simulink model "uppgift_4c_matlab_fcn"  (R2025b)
settings: Solver=VariableStepAuto  StartTime=0.0  StopTime=10.0  RelTol=1e-3
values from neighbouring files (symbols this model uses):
  AFs = 14.6    [Lektion_2.m]
  eta_vol = 0.8    [Lektion_2.m]
  m_dot_a_end = 18*1e-3    (= 0.018)    [Lektion_2.m]
  m_dot_a_start = 12*1e-3    (= 0.012)    [Lektion_2.m]
  m_dot_fi_start = m_dot_a_start/AFs    (= 0.000821917808219)    [Lektion_2.m]
  m_th_1 = 12/1000    (= 0.012)    [Lektion_2.m]
  n_cyl = 4    [Lektion_2.m]
  N_init = 3000/60    (= 50)    [Lektion_2.m]
  n_r = 2    [Lektion_2.m]
  R = 280    [Lektion_2.m]
  T_i = 320    [Lektion_2.m]
  tau_th = 1/0.1    (= 10)    [Lektion_2.m]
  V_d = 0.55/1e3    (= 0.00055)    [Lektion_2.m]
  V_i = 2/1e3    (= 0.002)    [Lektion_2.m]
undefined symbols (not defined in the file or in its folder): p_im

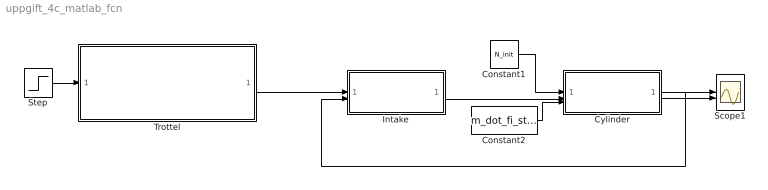
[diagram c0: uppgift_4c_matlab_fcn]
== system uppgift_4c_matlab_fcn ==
  Constant1 : Constant  Value=N_init
  Constant2 : Constant  Value=m_dot_fi_start
  Cylinder : Subsystem
  Intake : Subsystem
  Scope1 : Scope  NumInputPorts=2
  Step : Step  Time=3  Before=m_dot_a_start  After=m_dot_a_end  SampleTime=0
  Trottel : Subsystem
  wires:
  Cylinder/1(m_ac [kg/s]) -> Intake/2(m_ac [kg/s]), Scope1/1
  Step/1 -> Trottel/1(m_at,raf [kg/s])
  Trottel/1(m_at [kg/s]) -> Intake/1(m_at [kg/s])
  Cylinder/2(lambda_c [-]) -> Scope1/2
  Intake/1(p_im [Pa]) -> Cylinder/2(p_im [Pa])
  Constant1/1 -> Cylinder/1(N [rps])
  Constant2/1 -> Cylinder/3(m_fi [kg/s])

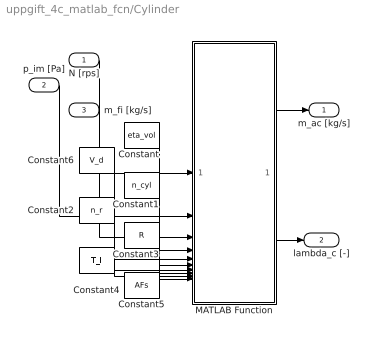
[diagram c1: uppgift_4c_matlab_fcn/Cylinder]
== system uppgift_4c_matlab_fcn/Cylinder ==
  N [rps] : Inport
  p_im [Pa] : Inport  Port=2
  m_fi [kg/s] : Inport  Port=3
  Constant : Constant  Value=eta_vol
  Constant1 : Constant  Value=n_cyl
  Constant2 : Constant  Value=n_r
  Constant3 : Constant  Value=R
  Constant4 : Constant  Value=T_i
  Constant5 : Constant  Value=AFs
  Constant6 : Constant  Value=V_d
  MATLAB Function : MATLAB Function  TreatAsAtomicUnit=on
  m_ac [kg/s] : Outport
  lambda_c [-] : Outport  Port=2
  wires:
  p_im [Pa]/1 -> MATLAB Function/2(p_im)
  m_fi [kg/s]/1 -> MATLAB Function/3(m_fi)
  MATLAB Function/2(lambda) -> lambda_c [-]/1
  MATLAB Function/1(m_ac) -> m_ac [kg/s]/1
  N [rps]/1 -> MATLAB Function/1(N)
  Constant/1 -> MATLAB Function/4(eta_vol)
  Constant5/1 -> MATLAB Function/10(AFs)
  Constant4/1 -> MATLAB Function/9(T)
  Constant3/1 -> MATLAB Function/8(R)
  Constant2/1 -> MATLAB Function/7(n_r)
  Constant1/1 -> MATLAB Function/6(n_cyl)
  Constant6/1 -> MATLAB Function/5(V_d)

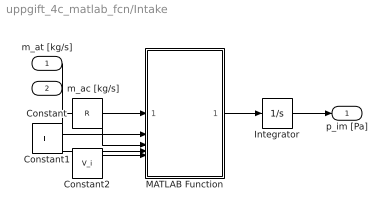
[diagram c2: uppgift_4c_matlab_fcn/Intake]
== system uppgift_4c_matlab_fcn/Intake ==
  m_at [kg/s] : Inport
  m_ac [kg/s] : Inport  Port=2
  Constant : Constant  Value=R
  Constant1 : Constant  Value=T_i
  Constant2 : Constant  Value=V_i
  Integrator : Integrator  InitialCondition=p_im
  MATLAB Function : MATLAB Function  TreatAsAtomicUnit=on
  p_im [Pa] : Outport
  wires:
  Integrator/1 -> p_im [Pa]/1
  MATLAB Function/1(y) -> Integrator/1
  m_ac [kg/s]/1 -> MATLAB Function/2(m_ac)
  m_at [kg/s]/1 -> MATLAB Function/1(m_at)
  Constant/1 -> MATLAB Function/3(R)
  Constant1/1 -> MATLAB Function/4(T)
  Constant2/1 -> MATLAB Function/5(V)

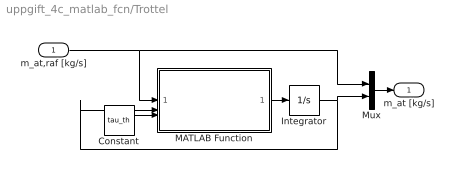
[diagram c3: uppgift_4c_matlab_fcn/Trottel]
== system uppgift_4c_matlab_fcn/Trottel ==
  m_at,raf [kg/s] : Inport
  Constant : Constant  Value=tau_th
  Integrator : Integrator  InitialCondition=m_th_1
  MATLAB Function : MATLAB Function  TreatAsAtomicUnit=on
  Mux : Mux  Inputs=2
  m_at [kg/s] : Outport
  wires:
  Integrator/1 -> MATLAB Function/2(actual), Mux/2
  Mux/1 -> m_at [kg/s]/1
  m_at,raf [kg/s]/1 -> MATLAB Function/1(ref), Mux/1
  MATLAB Function/1(alpha) -> Integrator/1
  Constant/1 -> MATLAB Function/3(tau)

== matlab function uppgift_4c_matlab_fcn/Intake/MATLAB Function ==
function y = fcn(m_at,m_ac,R,T,V)

y = u;

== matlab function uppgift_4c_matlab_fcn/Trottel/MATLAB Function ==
function alpha = fcn(ref, actual, tau)
error = ref - actual;

alpha =  error*tau;

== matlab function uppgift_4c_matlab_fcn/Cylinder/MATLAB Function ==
function [m_ac, lambda]= fcn(N, p_im, m_fi,eta_vol,V_d,n_cyl,n_r,R,T,AFs)

m_ac = eta_vol*N*p_im*V_d*n_cyl/(n_r*R*T);

lambda = m_ac/m_fi * 1/AFs;
